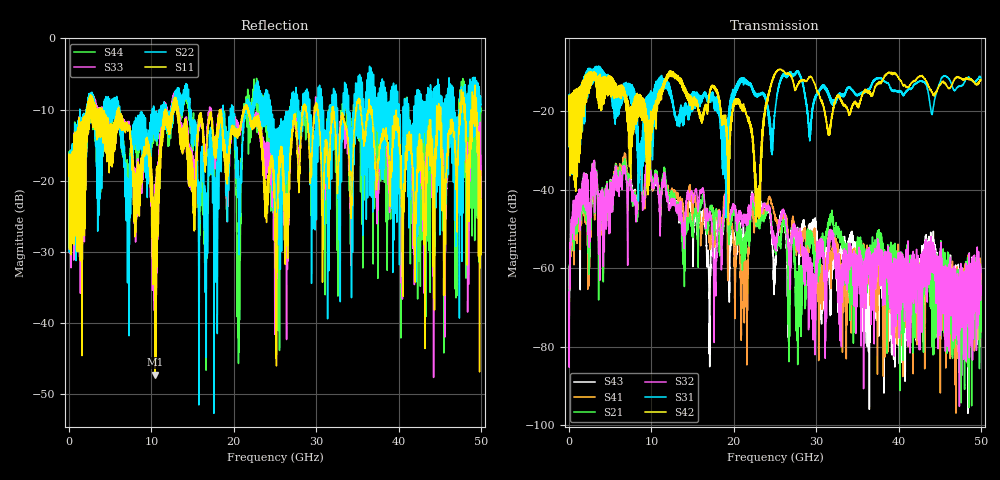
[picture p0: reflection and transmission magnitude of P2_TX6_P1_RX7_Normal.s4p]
!Keysight Technologies,N5225B,MY57041031,A.13.20.10
!Date: Friday, May 31, 2019 11:25:21
!Correction: S11(Full 4 Port(1,2,3,4))
!S12(Full 4 Port(1,2,3,4))
!S13(Full 4 Port(1,2,3,4))
!S14(Full 4 Port(1,2,3,4))
!S21(Full 4 Port(1,2,3,4))
!S22(Full 4 Port(1,2,3,4))
!S23(Full 4 Port(1,2,3,4))
!S24(Full 4 Port(1,2,3,4))
!S31(Full 4 Port(1,2,3,4))
!S32(Full 4 Port(1,2,3,4))
!S33(Full 4 Port(1,2,3,4))
!S34(Full 4 Port(1,2,3,4))
!S41(Full 4 Port(1,2,3,4))
!S42(Full 4 Port(1,2,3,4))
!S43(Full 4 Port(1,2,3,4))
!S44(Full 4 Port(1,2,3,4))
!S4P File: Measurements: <S11,S12,S13,S14>,
!<S21,S22,S23,S24>,
!<S31,S32,S33,S34>,
!<S41,S42,S43,S44>:
# Hz S  dB  R 50.0
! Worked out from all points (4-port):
!   5000 points, 10 MHz to 50 GHz, reference 50 ohm
!   strongest paths, dB at 10 MHz, 12.51 GHz, 25.01 GHz, 37.51 GHz, 50 GHz:
!     S42: -19.6, -9.9, -10.6, -12.7, -11.8
!     S31: -19.4, -16.8, -20.0, -11.7, -11.4
!     S32: -66.0, -42.9, -53.7, -56.2, -64.9
!     S21: -59.2, -41.2, -54.4, -52.5, -76.0
!     S41: -59.9, -40.0, -46.7, -63.7, -69.1
!     S43: -68.7, -42.3, -59.1, -62.2, -68.2
!   lowest |S11| = -47.3 dB at 10.41 GHz (marker M1), VSWR 1.01, Z = 50 - j0.431 ohm
!   |S11| at or under -10 dB: 6.028 GHz to 11.67 GHz (5.642 GHz wide, 63.8 % of centre); 21.74 GHz to 28.38 GHz (6.638 GHz wide, 26.5 % of centre); 36.76 GHz to 44.63 GHz (7.868 GHz wide, 19.3 % of centre)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
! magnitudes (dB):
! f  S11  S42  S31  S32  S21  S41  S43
! 10 MHz  -19.3  -19.6  -19.4  -66.0  -59.2  -59.9  -68.7
! 1.82 GHz  -17.5  -21.3  -17.2  -35.6  -36.4  -36.7  -36.2
! 10.41 GHz  -47.3  -19.2  -14.9  -36.7  -35.8  -36.7  -37.2
! 16.96 GHz  -11.6  -16.5  -16.1  -46.3  -47.6  -50.5  -62.0
! 22.93 GHz  -11.2  -39.8  -16.2  -46.8  -48.1  -45.5  -43.0
! 25.43 GHz  -21.7  -9.4  -13.7  -50.1  -52.4  -50.0  -51.0
! 50 GHz  -22.6  -11.8  -11.4  -64.9  -76.0  -69.1  -68.2
